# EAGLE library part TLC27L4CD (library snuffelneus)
OPERATION AMPLIFIERS
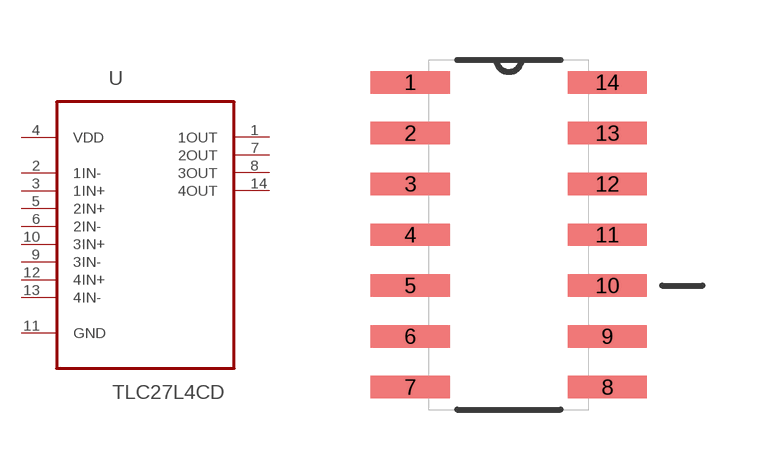
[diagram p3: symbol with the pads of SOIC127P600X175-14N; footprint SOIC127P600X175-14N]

Designator prefix U

## TLC27L4CD (MPN: TLC27L4CD; OC_FARNELL: 1106127; OC_NEWARK: 67K1259; PACKAGE: SOIC-14; SUPPLIER: Texas Instruments)  [SOIC127P600X175-14N]
1  1OUT  out
2  1IN-  in
3  1IN+  in
4  VDD  pwr
5  2IN+  in
6  2IN-  in
7  2OUT  out
8  3OUT  out
9  3IN-  in
10  3IN+  in
11  GND  pas
12  4IN+  in
13  4IN-  in
14  4OUT  out

## Footprint SOIC127P600X175-14N (pad centres in mm)
smd 1.981 x 0.559: 1 -2.464,3.81; 2 -2.464,2.54; 3 -2.464,1.27; 4 -2.464,0; 5 -2.464,-1.27; 6 -2.464,-2.54; 7 -2.464,-3.81; 8 2.464,-3.81; 9 2.464,-2.54; 10 2.464,-1.27; 11 2.464,0; 12 2.464,1.27; 13 2.464,2.54; 14 2.464,3.81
